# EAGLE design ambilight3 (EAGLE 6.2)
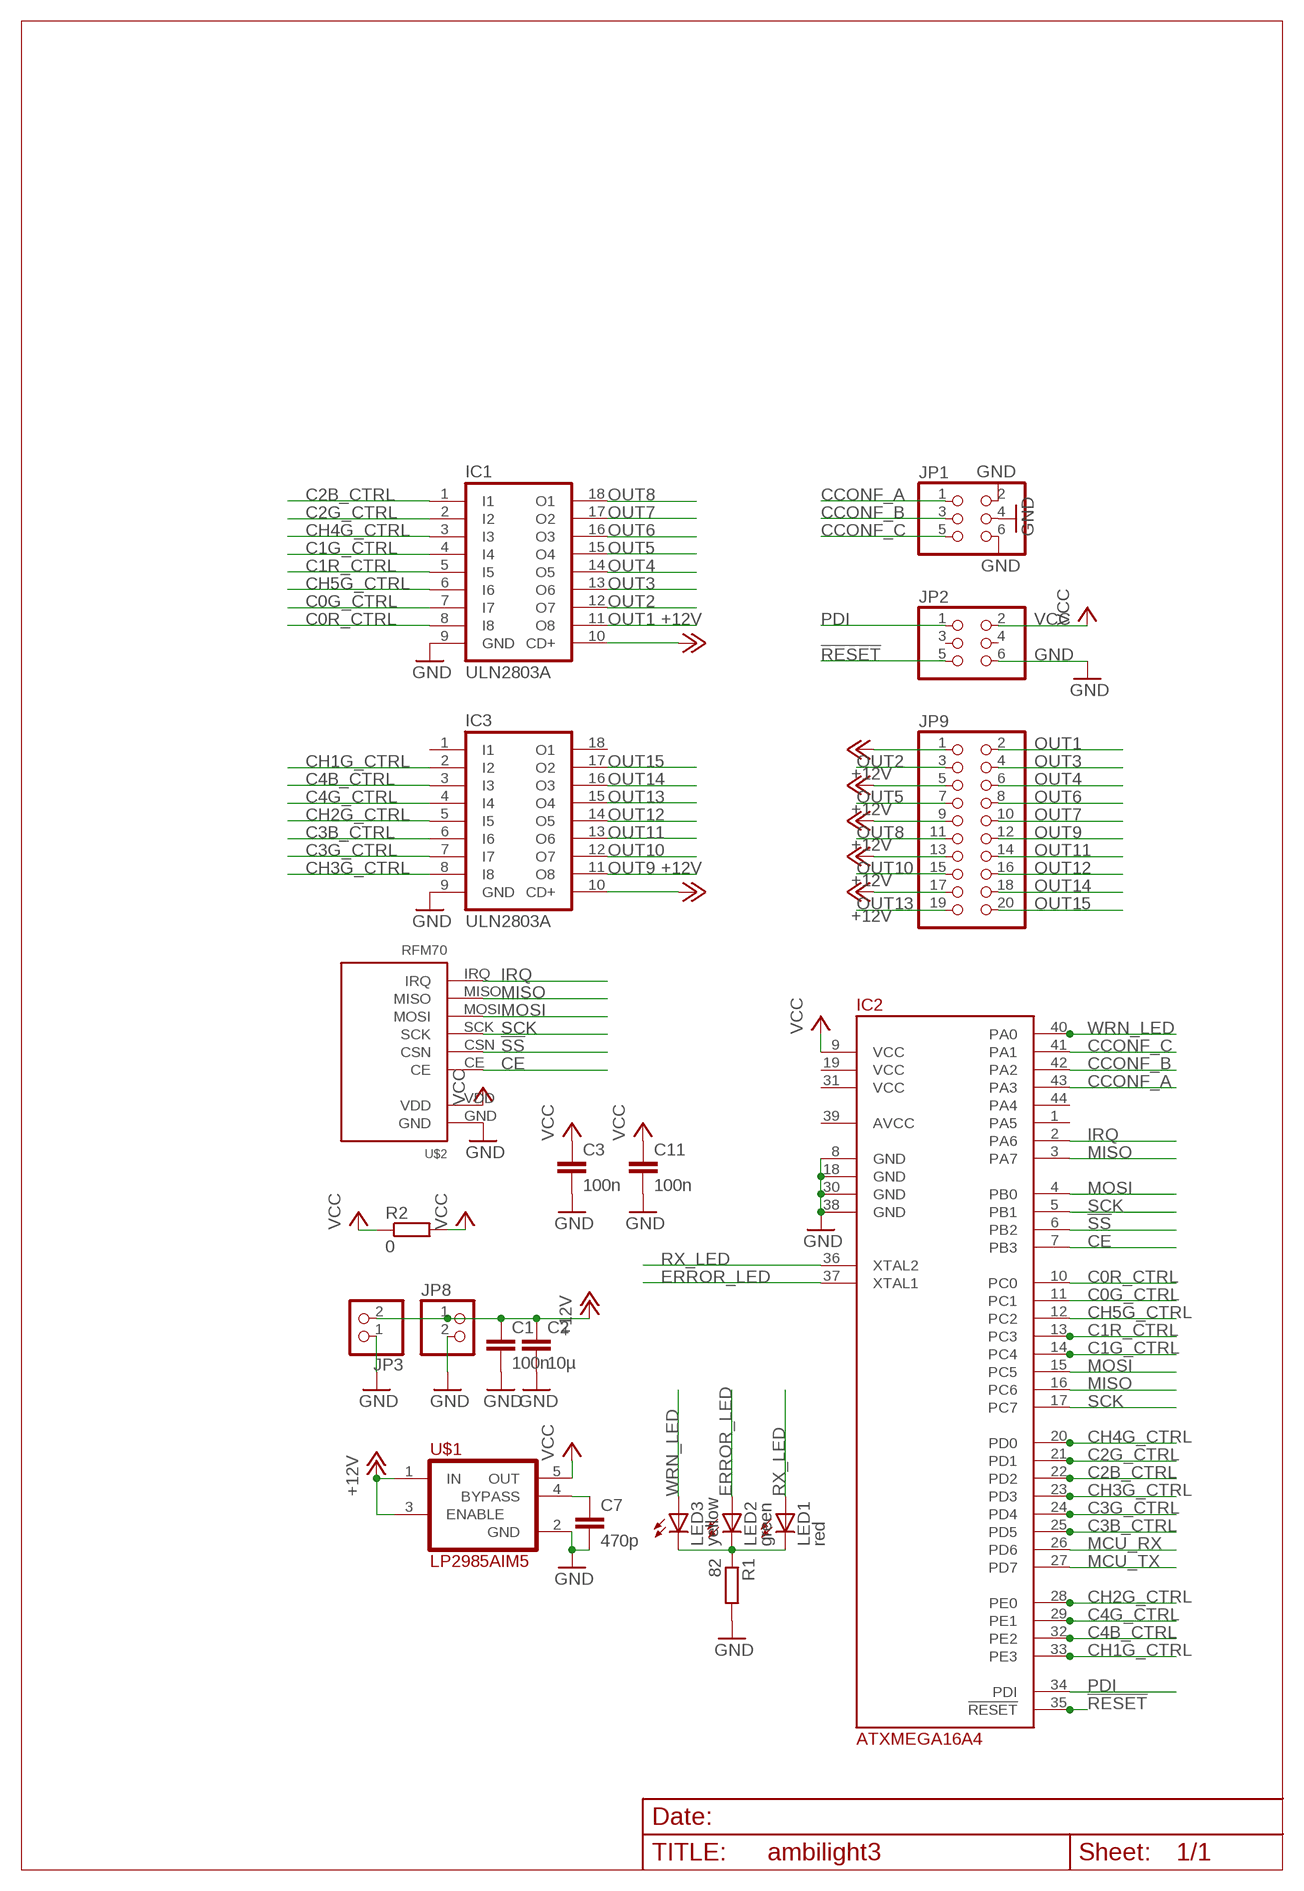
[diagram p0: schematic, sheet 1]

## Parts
C1  100n  C-EUC1206K  [C1206K]
C2  10µ  C-EUC1206K  [C1206K]
C3  100n  C-EUC1206K  [C1206K]
C7  470p  C-EUC1206K  [C1206K]
C11  100n  C-EUC1206K  [C1206K]
IC1  ULN2803A  ULN2803ADW  [SO18W]
IC2  ATXMEGA16A4  ATXMEGA_A4  [TQFP44]
IC3  ULN2803A  ULN2803ADW  [SO18W]
JP1  PINHD-2X03_2.54-SMD  [2X03SMD]
JP2  PINHD-2X03_2.54-SMD  [2X03SMD]
JP3  PINHD-1X02_2.54-SMD-90°  [1X02SMD/90]
JP8  PINHD-1X02_2.54-SMD-90°  [1X02SMD/90]
JP9  PINHD-2X10_2.54-SMD  [2X10SMD]
LED1  red  LEDCHIPLED_1206  [CHIPLED_1206]
LED2  green  LEDCHIPLED_1206  [CHIPLED_1206]
LED3  yellow  LEDCHIPLED_1206  [CHIPLED_1206]
R1  82  R-EU_M1206  [M1206]
R2  0  R-EU_M1206  [M1206]
U$1  LP2985AIM5  [SOT25]
U$2  RFM70  [RFM70]

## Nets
!RESET: IC2.35(!RESET) JP2.5
!SS: IC2.6(PB2) U$2.CSN
+12V: C1.1 C2.1 IC1.10(CD+) IC3.10(CD+) JP3.2 JP8.1 JP9.1 JP9.5 JP9.9 JP9.13 JP9.17 U$1.1(IN) U$1.3(ENABLE)
C0G_CTRL: IC1.7(I7) IC2.11(PC1)
C0R_CTRL: IC1.8(I8) IC2.10(PC0)
C1G_CTRL: IC1.4(I4) IC2.14(PC4)
C1R_CTRL: IC1.5(I5) IC2.13(PC3)
C2B_CTRL: IC1.1(I1) IC2.22(PD2)
C2G_CTRL: IC1.2(I2) IC2.21(PD1)
C3B_CTRL: IC2.25(PD5) IC3.6(I6)
C3G_CTRL: IC2.24(PD4) IC3.7(I7)
C4B_CTRL: IC2.32(PE2) IC3.3(I3)
C4G_CTRL: IC2.29(PE1) IC3.4(I4)
CCONF_A: IC2.43(PA3) JP1.1
CCONF_B: IC2.42(PA2) JP1.3
CCONF_C: IC2.41(PA1) JP1.5
CE: IC2.7(PB3) U$2.CE
CH1G_CTRL: IC2.33(PE3) IC3.2(I2)
CH2G_CTRL: IC2.28(PE0) IC3.5(I5)
CH3G_CTRL: IC2.23(PD3) IC3.8(I8)
CH4G_CTRL: IC1.3(I3) IC2.20(PD0)
CH5G_CTRL: IC1.6(I6) IC2.12(PC2)
ERROR_LED: IC2.37(XTAL1) LED2.A
GND: C1.2 C2.2 C3.2 C7.2 C11.2 IC1.9(GND) IC2.8(GND) IC2.18(GND) IC2.30(GND) IC2.38(GND) IC3.9(GND) JP1.2 JP1.4 JP1.6 JP2.6 JP3.1 JP8.2 R1.2 U$1.2(GND) U$2.GND
IRQ: IC2.2(PA6) U$2.IRQ
MCU_RX: IC2.26(PD6)
MCU_TX: IC2.27(PD7)
MISO: IC2.3(PA7) IC2.16(PC6) U$2.MISO
MOSI: IC2.4(PB0) IC2.15(PC5) U$2.MOSI
N$1: LED1.C LED2.C LED3.C R1.1
N$10: C7.1 U$1.4(BYPASS)
OUT1: IC1.11(O8) JP9.2
OUT2: IC1.12(O7) JP9.3
OUT3: IC1.13(O6) JP9.4
OUT4: IC1.14(O5) JP9.6
OUT5: IC1.15(O4) JP9.7
OUT6: IC1.16(O3) JP9.8
OUT7: IC1.17(O2) JP9.10
OUT8: IC1.18(O1) JP9.11
OUT9: IC3.11(O8) JP9.12
OUT10: IC3.12(O7) JP9.15
OUT11: IC3.13(O6) JP9.14
OUT12: IC3.14(O5) JP9.16
OUT13: IC3.15(O4) JP9.19
OUT14: IC3.16(O3) JP9.18
OUT15: IC3.17(O2) JP9.20
PDI: IC2.34(PDI) JP2.1
RX_LED: IC2.36(XTAL2) LED1.A
SCK: IC2.5(PB1) IC2.17(PC7) U$2.SCK
VCC: C3.1 C11.1 IC2.9(VCC) JP2.2 R2.1 R2.2 U$1.5(OUT) U$2.VDD
WRN_LED: IC2.40(PA0) LED3.A
Unconnected: IC2.1(PA5) IC2.44(PA4) IC3.1(I1) IC3.18(O1) JP2.3 JP2.4

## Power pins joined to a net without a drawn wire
AVCC: IC2.39(AVCC)
VCC: IC2.19(VCC) IC2.31(VCC)

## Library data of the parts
C1-C3 C7 C11 = rcl:C-EU: CAPACITOR, European symbol
IC1 IC3 = uln-udn:ULN2803A: DRIVER ARRAY
IC2 = atmel_xmega:ATXMEGA_A4
JP1 JP2 = pinhead-2:PINHD-2X03: PIN HEADER
JP3 JP8 = pinhead-2:PINHD-1X02: PIN HEADER
JP9 = pinhead-2:PINHD-2X10: PIN HEADER
LED1-LED3 = led:LED: LED
R1 R2 = rcl:R-EU_: RESISTOR, European symbol
U$1 = v-reg:LP2985AIM5
U$2 = rfm70:RFM70: RFM70 2.4 Ghz Funkmodul Autor: Daniel Weber Website: http://projects.web4clans.com Email: daniel.weber@web4clans.com

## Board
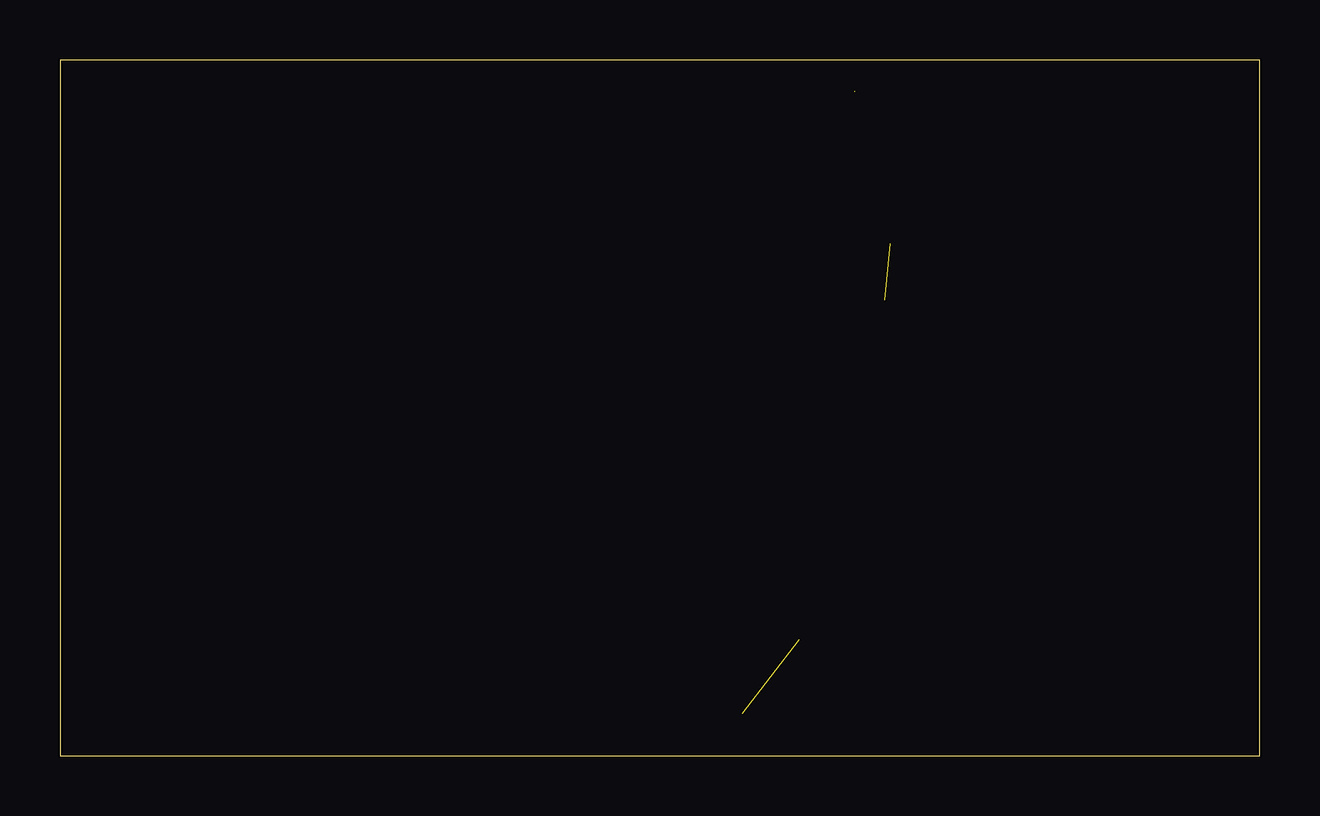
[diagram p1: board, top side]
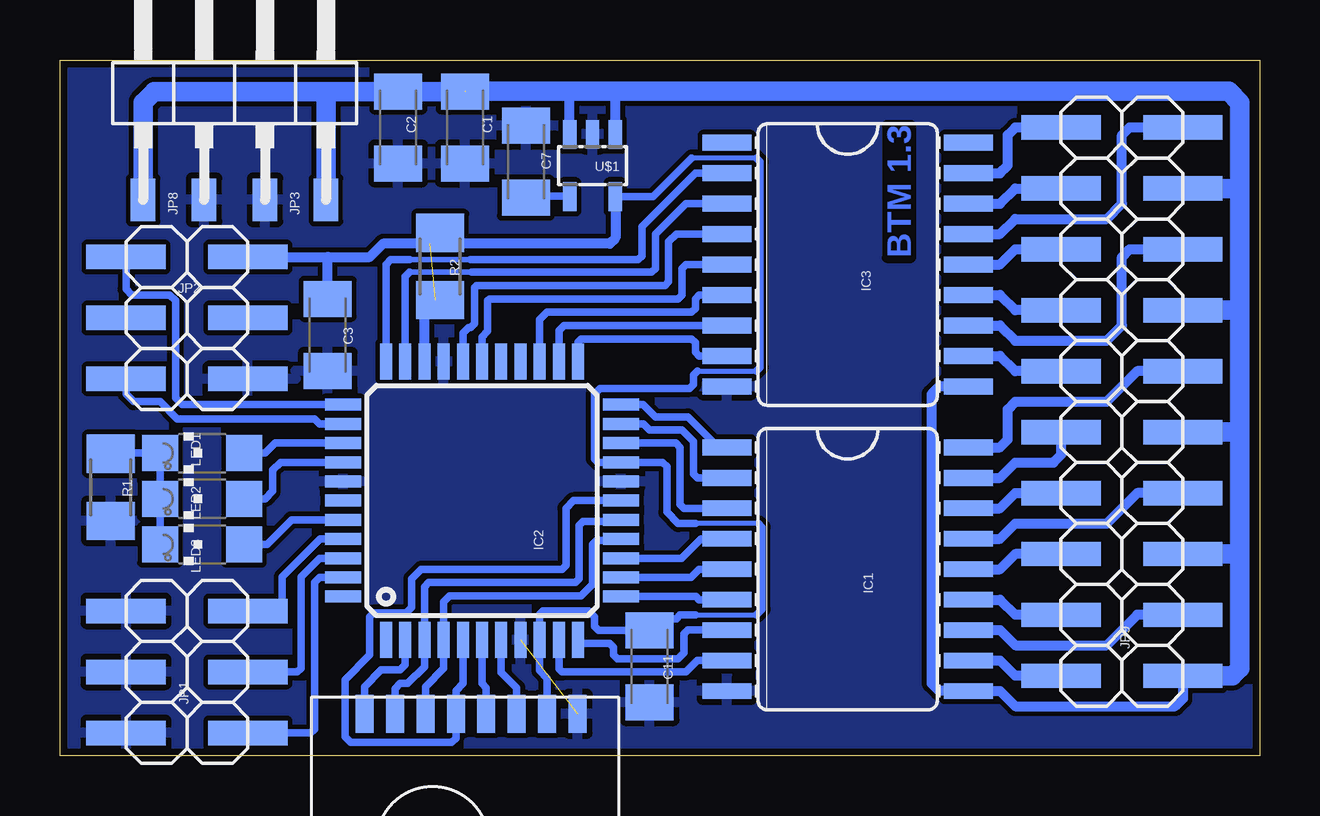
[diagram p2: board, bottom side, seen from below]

Size 50 x 29 mm. Coordinates in mm from the lower left corner, seen from the top.
Outline: 0,0 50,0 50,29 0,29 0,0
Copper layers (1*16): Top 0.035mm / dielectric 1.5mm / Bottom 0.035mm
Design rules: minimum track width 8mil, minimum drill 24mil, track to track 8mil, track to pad 8mil, pad to pad 8mil, via to via 8mil, smd to smd 8mil, copper to edge 12mil, drill to drill 8mil, minimum pad ring 10mil, minimum via ring 8mil, stop-mask expansion 4mil, vias tented up to drill 0mil, thermal gap 10mil

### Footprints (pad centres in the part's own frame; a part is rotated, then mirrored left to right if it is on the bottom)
C1206K = smd 1.5 x 2: 1 -1.5,0; 2 1.5,0
SO18W = smd 0.66 x 2.032: 1 -5.08,-5.029; 2 -3.81,-5.029; 3 -2.54,-5.029; 4 -1.27,-5.029; 5 0,-5.029; 6 1.27,-5.029; 7 2.54,-5.029; 8 3.81,-5.029; 9 5.08,-5.029; 10 5.08,5.029; 11 3.81,5.029; 12 2.54,5.029; 13 1.27,5.029; 14 0,5.029; 15 -1.27,5.029; 16 -2.54,5.029; 17 -3.81,5.029; 18 -5.08,5.029
TQFP44 = smd 1.5 x 0.5: 1 -5.8,4; 2 -5.8,3.2; 3 -5.8,2.4; 4 -5.8,1.6; 5 -5.8,0.8; 6 -5.8,0; 7 -5.8,-0.8; 8 -5.8,-1.6; 9 -5.8,-2.4; 10 -5.8,-3.2; 11 -5.8,-4; 23 5.8,-4; 24 5.8,-3.2; 25 5.8,-2.4; 26 5.8,-1.6; 27 5.8,-0.8; 28 5.8,0; 29 5.8,0.8; 30 5.8,1.6; 31 5.8,2.4; 32 5.8,3.2; 33 5.8,4 | smd 0.5 x 1.5: 12 -4,-5.8; 13 -3.2,-5.8; 14 -2.4,-5.8; 15 -1.6,-5.8; 16 -0.8,-5.8; 17 0,-5.8; 18 0.8,-5.8; 19 1.6,-5.8; 20 2.4,-5.8; 21 3.2,-5.8; 22 4,-5.8; 34 4,5.8; 35 3.2,5.8; 36 2.4,5.8; 37 1.6,5.8; 38 0.8,5.8; 39 0,5.8; 40 -0.8,5.8; 41 -1.6,5.8; 42 -2.4,5.8; 43 -3.2,5.8; 44 -4,5.8
2X03SMD = smd 1.016 x 3.302: 1 -1.27,-3.81; 2 -1.27,1.27; 3 1.27,-3.81; 4 1.27,1.27; 5 3.81,-3.81; 6 3.81,1.27
1X02SMD/90 = smd 1.016 x 1.778: 1 -1.27,-5.08; 2 1.27,-5.08
2X10SMD = smd 1.016 x 3.302: 1 -1.27,-3.81; 2 -1.27,1.27; 3 1.27,-3.81; 4 1.27,1.27; 5 3.81,-3.81; 6 3.81,1.27; 7 6.35,-3.81; 8 6.35,1.27; 9 8.89,-3.81; 10 8.89,1.27; 11 11.43,-3.81; 12 11.43,1.27; 13 13.97,-3.81; 14 13.97,1.27; 15 16.51,-3.81; 16 16.51,1.27; 17 19.05,-3.81; 18 19.05,1.27; 19 21.59,-3.81; 20 21.59,1.27
CHIPLED_1206 = smd 1.5 x 1.5: A 0,-1.75; C 0,1.75
M1206 = smd 1.6 x 2: 1 -1.4,0; 2 1.4,0
SOT25 = smd 0.55 x 1.2: 1 -0.95,-1.3; 2 0,-1.3; 3 0.95,-1.3; 4 0.95,1.3; 5 -0.95,1.3
RFM70 = smd 0.75 x 1.6: CE -2.16,-7.7; CSN -0.89,-7.7; GND -4.7,-7.7; IRQ 4.19,-7.7; MISO 2.92,-7.7; MOSI 1.65,-7.7; SCK 0.38,-7.7; VDD -3.43,-7.7

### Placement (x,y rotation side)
C1  33.12,26.18 270 bottom
C2  35.9,26.18 270 bottom
C3  38.83,17.53 270 bottom
C7  30.58,24.76 90 bottom
C11  25.42,3.72 270 bottom
IC1  17.16,7.77 270 bottom
IC2  32.41,10.63 90 bottom
IC3  17.16,20.47 270 bottom
JP1  45.98,2.21 90 bottom
JP2  43.44,19.52 270 bottom
JP3  40.18,28.25 0 bottom
JP8  45.26,28.25 0 bottom
JP9  7,4.59 90 bottom
LED1  44.07,12.61 90 bottom
LED2  44.07,10.71 90 bottom
LED3  44.07,8.8 90 bottom
R1  47.88,11.18 270 bottom
R2  34.15,20.39 90 bottom
U$1  27.8,24.6 180 bottom
U$2  33.12,-5.96 180 bottom

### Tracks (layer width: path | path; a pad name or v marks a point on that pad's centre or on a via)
!RESET
  Bottom 0.305: IC2.35 39.18,13.83 39.39,14.04 45.1,14.04 45.82,14.76 46.93,14.76 47.25,15.07 JP2.5
!SS
  Bottom 0.305: U$2.CSN 32.23,2.83 32.41,3.01 IC2.6
+12V  (1 unrouted)
  Bottom 0.406: IC3.10 13.36,15.39 13.67,15.07 13.67,3.01 13.36,2.69 IC1.10 10.81,2.69 10.18,2.06 3.51,2.06 3.19,2.37 JP9.1 | U$1.3 28.75,27.69 | U$1.1 26.85,27.69
  Bottom 0.813: JP9.1 1.13,3.33 0.81,3.64 0.81,8.4 | 0.81,8.4 0.81,13.48 | 0.81,13.48 0.81,18.57 | 0.81,18.57 0.81,23.64 | JP9.5 0.81,8.4 | JP9.9 0.81,13.48 | JP9.13 0.81,18.57 | JP9.17 0.81,23.64 | 0.81,23.64 0.81,27.22 1.29,27.69 26.85,27.69 28.75,27.69 | 28.75,27.69 arc-90 28.75,27.69 | 28.75,27.69 33.12,27.69 | C1.1 C2.1 38.91,27.68 | 38.91,27.68 46.06,27.68 46.53,27.22 JP8.1 | 38.91,27.68 JP3.2
C0G_CTRL
  Bottom 0.305: IC1.7 23.83,5.23 23.99,5.07 23.99,4.28 24.23,4.04 26.77,4.04 26.93,4.2 26.93,4.52 27.09,4.67 28.36,4.67 28.41,4.72 IC2.11
C0R_CTRL
  Bottom 0.305: IC1.8 23.44,3.96 23.91,3.48 29.07,3.48 29.2,3.62 IC2.10
C1G_CTRL
  Bottom 0.305: IC2.14 24.09,8.23 23.28,9.04 IC1.4
C1R_CTRL
  Bottom 0.305: IC2.13 23.7,7.43 23.36,7.77 IC1.5
C2B_CTRL
  Bottom 0.305: IC2.22 25.69,14.63 25.18,14.12 23.83,14.12 22.56,12.85 IC1.1
C2G_CTRL
  Bottom 0.305: IC1.2 23.44,11.58 23.59,11.74 23.59,13.09 24.07,13.56 25.42,13.56 25.68,13.83 IC2.21
C3B_CTRL
  Bottom 0.305: IC3.6 23.36,19.2 23.52,19.04 23.52,18.64 23.67,18.49 29.71,18.49 30,18.19 IC2.25
C3G_CTRL
  Bottom 0.305: IC3.7 28.99,17.93 29.2,17.72 IC2.24
C4B_CTRL
  Bottom 0.229: 32.84,20.15 35.42,20.15
  Bottom 0.305: IC2.32 35.6,19.97 35.42,20.15 | 32.84,20.15 25.34,20.15 25.18,20.31 25.18,21.74 23.91,23.01 IC3.3
C4G_CTRL
  Bottom 0.305: IC3.4 24.31,21.74 24.63,21.42 24.63,19.76 24.79,19.6 32.64,19.6 32.72,19.52 32.72,18.01 32.88,17.85 32.96,17.85 33.2,17.61 IC2.29
CCONF_A
  Bottom 0.305: IC2.43 39.18,7.43 39.39,7.21 39.39,1.1 39.55,0.94 JP1.1
CCONF_B
  Bottom 0.305: JP1.3 40.1,3.48 39.95,3.64 39.95,7.45 39.17,8.23 IC2.42
CCONF_C
  Bottom 0.305: IC2.41 39.16,9.03 40.74,7.45 40.74,6.02 JP1.5
CE
  Bottom 0.305: U$2.CE 30.96,2.83 31.61,3.48 IC2.7
CH1G_CTRL
  Bottom 0.229: 35.42,20.67 32.88,20.67
  Bottom 0.305: IC2.33 36.41,20.48 36.22,20.67 35.42,20.67 | 32.88,20.67 25.9,20.67 25.74,20.83 25.74,22.06 23.52,24.28 IC3.2
CH2G_CTRL
  Bottom 0.305: IC3.5 23.91,20.47 24.07,20.31 24.07,19.2 24.23,19.04 32.09,19.04 32.17,18.96 32.17,17.69 32.41,17.45 IC2.28
CH3G_CTRL
  Bottom 0.305: IC3.8 23.36,16.66 23.52,16.82 23.52,17.22 23.67,17.37 28.28,17.37 28.41,17.25 IC2.23
CH4G_CTRL
  Bottom 0.305: IC1.3 23.99,10.31 24.15,10.47 24.15,12.85 24.33,13.03 IC2.20
CH5G_CTRL
  Bottom 0.305: IC1.6 23.36,6.5 23.48,6.63 IC2.12
ERROR_LED
  Bottom 0.305: LED2.A 41.45,10.71 41.14,11.02 41.14,11.9 40.81,12.23 IC2.37
GND  (1 unrouted)
  pour Bottom: 0,29 50,29 50,0 0,0
IRQ
  Bottom 0.305: IC2.2 35.6,3.78 35.82,3.56 36.61,3.56 37.31,2.87 U$2.IRQ
MISO
  Bottom 0.305: U$2.MISO 36.04,2.79 35.82,3.01 35.5,3.01 34.8,3.7 IC2.3 34.8,7.04 34.63,7.21 28.52,7.21 28.36,7.37 28.36,9.6 28.2,9.75 26.61,9.75 26.61,9.76 IC2.16
MOSI
  Bottom 0.305: U$2.MOSI 34.77,2.87 34.01,3.63 IC2.4 34.01,6.41 33.75,6.66 28.28,6.66 27.8,7.13 27.8,8.8 27.64,8.96 26.77,8.96 26.7,9.03 IC2.15
N$1
  Bottom 0.305: LED3.C LED2.C LED1.C 47.85,12.61 R1.1
N$10
  Bottom 0.305: U$1.4 arc-90 28.78,23.33 30.33,23.33 arc90 C7.1
OUT1
  Bottom 0.406: IC1.11 10.81,3.96 10.18,3.33 JP9.2
OUT2
  Bottom 0.406: IC1.12 10.81,5.23 10.18,4.59 6.37,4.59 5.1,5.87 JP9.3
OUT3
  Bottom 0.406: IC1.13 10.81,6.5 10.18,5.87 JP9.4
OUT4
  Bottom 0.406: IC1.14 10.81,7.77 10.18,8.4 JP9.6
OUT5
  Bottom 0.406: IC1.15 10.81,9.04 10.18,9.68 6.37,9.68 5.1,10.95 JP9.7
OUT6
  Bottom 0.406: IC1.16 10.81,10.31 10.18,10.95 JP9.8
OUT7
  Bottom 0.406: IC1.17 10.81,11.58 10.18,12.21 8.59,12.21 8.28,12.53 JP9.10
OUT8
  Bottom 0.406: IC1.18 10.81,12.85 10.5,13.17 10.5,14.44 10.18,14.76 6.37,14.76 5.1,16.02 JP9.11
OUT9
  Bottom 0.406: IC3.11 10.81,16.66 10.18,16.02 JP9.12
OUT10
  Bottom 0.406: IC3.12 10.81,17.93 10.18,17.3 6.37,17.3 5.74,17.93 5.74,20.79 5.42,21.11 JP9.15
OUT11
  Bottom 0.406: IC3.13 10.81,19.2 10.18,18.57 JP9.14
OUT12
  Bottom 0.406: IC3.14 10.81,20.47 10.18,21.11 JP9.16
OUT13
  Bottom 0.406: IC3.15 10.81,21.74 10.18,22.38 6.37,22.38 5.74,23.01 5.74,25.87 5.42,26.18 JP9.19
OUT14
  Bottom 0.406: IC3.16 10.81,23.01 10.18,23.64 JP9.18
OUT15
  Bottom 0.406: IC3.17 10.81,24.28 10.5,24.6 10.5,25.87 10.18,26.18 JP9.20
PDI
  Bottom 0.305: IC2.34 44.9,14.63 45.18,14.91 45.18,18.96 45.42,19.2 47.01,19.2 47.25,19.44 JP2.1
RX_LED
  Bottom 0.305: LED1.A 41.45,12.61 41.04,13.03 IC2.36
SCK
  Bottom 0.305: IC2.5 33.2,3 33.5,2.71 U$2.SCK 33.5,0.72 33.67,0.55 37.88,0.55 38.12,0.79 38.12,3.17 37.09,4.2 37.09,5.79 36.93,5.94 35.58,5.94 35.34,6.18 35.34,7.37 34.95,7.77 29.07,7.77 28.91,7.93 28.91,10.31 28.59,10.63 IC2.17
VCC  (1 unrouted)
  Bottom 0.203: 23.44,16.02 20.98,16.02 | 20.98,24.91 23.67,24.91 | 23.52,5.87 20.98,5.87 | 20.9,9.68 23.52,9.68
  Bottom 0.305: U$2.VDD 29.69,3.23 30,3.54 IC2.9 30,5.88 29.86,6.02 27.96,6.02 27.72,5.79 27.72,5.39 27.55,5.22 C11.1 24.94,5.71 24.31,5.71 24.15,5.87 23.52,5.87 | 20.98,5.87 20.74,6.1 20.74,9.52 20.9,9.68 | 23.44,16.02 23.59,15.87 23.59,15.47 23.75,15.31 27.48,15.31 27.72,15.07 27.72,12.37 27.58,12.23 IC2.19 24.88,12.23 24.71,12.06 24.71,10.15 24.23,9.68 23.52,9.68 | 20.98,16.02 20.82,16.18 20.82,24.76 20.98,24.91 | 23.67,24.91 25.29,23.3 U$1.5
  Bottom 0.406: JP2.2 38.83,20.79 | 38.83,20.79 37.09,20.79 36.53,21.34 34.6,21.34 R2.2 33.7,21.34 27.09,21.34 26.85,21.58 U$1.5 | IC2.31 34.8,18.55 34.36,18.99 R2.1 | C3.1 38.83,20.79
WRN_LED
  Bottom 0.305: LED3.A 41.37,8.8 40.35,9.83 IC2.40

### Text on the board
Bottom: BTM 1.3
